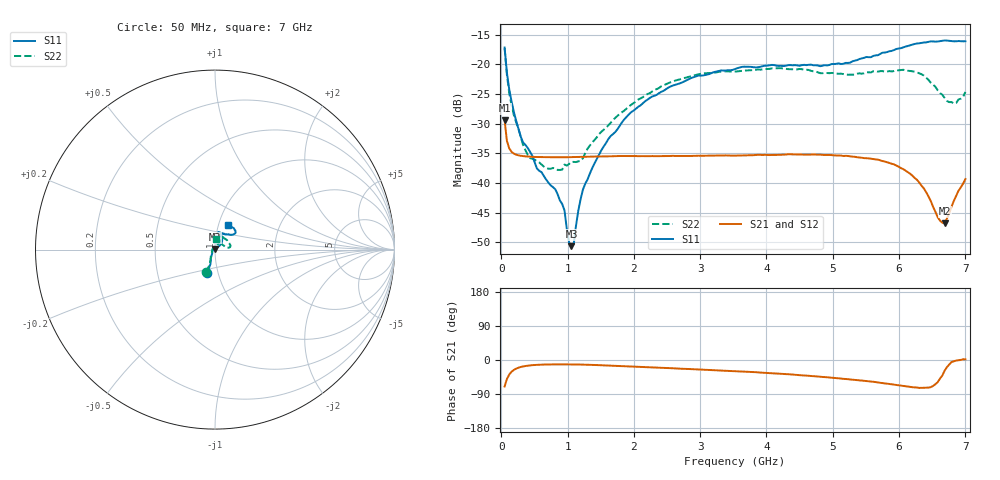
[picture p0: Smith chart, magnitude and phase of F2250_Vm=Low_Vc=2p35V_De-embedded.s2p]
! Integrated Device Technology
! Corporate Headquarters
! 6024 Silver Creek Valley Road
! San Jose, CA 95138  USA
! Phone:  1-408-284-8200
! Toll Free:  1-800-223-1366
! Webpage:  http://www.idt.com/
! Timing and RF Division
! 515 Groton Road, Suite 102
! Westford, MA 01886-6024
! Device:  F2250
! Description: Voltage Variable RF Attenuator
! Frequency:  50.0 -  6000.00 MHz
! Package:  3x3 mm Thin QFN Plastic Package: 16 pin
! Ports:  2 RF, 3 DC
!  Pin  1  = GND
!  Pin  2  = NC
!  Pin  3  = RF1  = Port 1
!  Pin  4  = NC
!  Pin  5  = GND
!  Pin  6  = GND
!  Pin  7  = GND
!  Pin  8  = GND
!  Pin  9  = NC
!  Pin 10  = RF2  = Port 2
!  Pin 11  = NC
!  Pin 12  = GND
!  Pin 13  = GND
!  Pin 14  = VCNTRL
!  Pin 15  = VDD
!  Pin 16  = VMODE
! Vcntrl:  2.350 Volts
! Vmode:  +0.000 Volts
! Vdd:  +3.30  Volts
! Current:  1.176 mA
! Data:  The device was measured on a the F2250 evaluation board which has
!  individual transmission lines to the RF pins.  Data was collected
!  using a calibrated network analyzer.  The evaluation board was
!  de-embedded using a TRL calibration technique.
!  The reference plane is the edge of the package pin.
! Misc:  SN 10
!  Action Tracker AT0258
! Date Measured:  2014-11-26
! Date:  2015-10-15  MJV
! Note:
!  Integrated Device Technology supplies this data as a sample of measured
!  data at the package pin for this product.  Your particular data for this
!  product may vary.
!  Data was taken at 25 degrees C.
!  Integrated Device Technology reserves the right to change this data at anytime.
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# GHz S dB R 50
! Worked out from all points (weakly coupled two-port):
!   201 points, 50 MHz to 7 GHz, reference 50 ohm
!   highest |S21| = -29.41 dB at 50 MHz (marker M1); lowest = -46.8 dB at 6.687 GHz (marker M2)
!   lowest |S11| = -50.6 dB at 1.058 GHz (marker M3), VSWR 1.01, Z = 49.8 + j0.245 ohm
!   |S11| at or under -10 dB: start of sweep to end of sweep
!   |S22| runs from -37.8 to -17.3 dB; largest |S21 - S12| = 5.3e-05
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0.05  -17.18 -108.6  -29.41 -69.8  -29.41 -69.7  -17.30 -110.9
0.08475  -21.44 -107.4  -32.91 -50.3  -32.91 -50.3  -21.78 -110.0
0.15425  -26.23 -116.6  -34.74 -31.1  -34.74 -31.1  -26.87 -121.9
0.29325  -32.20 -127.7  -35.42 -18.4  -35.42 -18.4  -32.23 -136.9
0.3975  -34.08 -141.8  -35.54 -15.0  -35.54 -15.0  -35.25 -159.9
0.91875  -43.54 158.1  -35.67 -11.5  -35.67 -11.5  -37.74 132.4
0.9535  -44.63 169.8  -35.67 -11.6  -35.66 -11.5  -36.89 130.3
1.023  -50.05 143.8  -35.66 -11.6  -35.66 -11.6  -36.79 114.6
1.05775  -50.64 123.3  -35.65 -11.6  -35.65 -11.6  -36.45 109.3
1.0925  -50.34 90.8  -35.65 -11.7  -35.64 -11.7  -36.45 104.6
1.162  -44.62 57.0  -35.62 -11.9  -35.62 -11.9  -36.35 94.0
1.2315  -41.11 44.4  -35.59 -12.1  -35.59 -12.1  -35.84 84.4
1.6485  -32.11 41.9  -35.51 -14.7  -35.50 -14.7  -29.88 63.8
1.96125  -28.05 42.2  -35.45 -17.2  -35.45 -17.2  -26.82 56.3
2.37825  -24.87 47.3  -35.47 -20.3  -35.46 -20.3  -24.00 56.4
3.525  -20.80 72.5  -35.39 -29.6  -35.39 -29.6  -21.23 74.6
4.7065  -20.17 72.3  -35.19 -42.5  -35.19 -42.6  -21.19 72.2
5.85325  -17.82 40.5  -36.62 -63.3  -36.63 -63.3  -21.15 22.8
6.27025  -16.50 40.1  -39.47 -72.6  -39.48 -72.6  -21.37 9.4
6.68725  -15.99 48.8  -46.82 -28.0  -46.80 -27.6  -25.68 28.2
6.861  -16.13 55.1  -42.17 -1.5  -42.13 -1.4  -26.52 57.9
7  -16.12 63.2  -39.34 1.7  -39.31 1.6  -24.66 83.2
